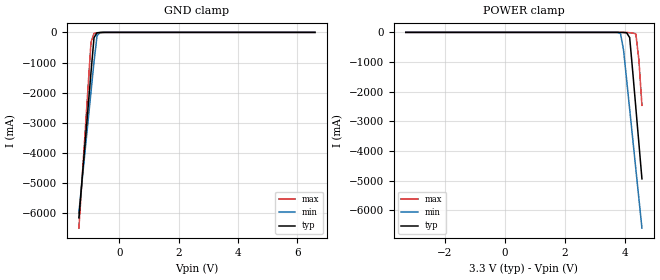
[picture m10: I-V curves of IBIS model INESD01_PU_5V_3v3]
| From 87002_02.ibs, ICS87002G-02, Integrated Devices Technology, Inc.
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[Model] INESD01_PU_5V_3v3
Model_type  Input
Polarity   Non-Inverting
Vinl = 0.8V
Vinh = 2.0V
|   typ   min   max
C_comp   2pF   1.5pF   2.5pF
|   typ   min   max
[Voltage range]  3.3V   3.15V   3.45V
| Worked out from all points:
|   GND clamp passes 1 mA (typ) near -0.55 V on its own axis
[GND_clamp]
|Voltage   I(typ)   I(min)   I(max)
-1.361V   -6.144A    -5.981A    -6.488A
-952.6mV  -1.327A    -1.975A    -329.1mA
-850.5mV  -175.3mA   -975.1mA   -32.14mA
-748.5mV  -12.69mA   -105.5mA   -18.41mA
-646.4mV  -3.879mA   -5.373mA   -8.361mA
6.6V      64.3uA     69.07uA    57.85uA
[POWER_clamp]
|Voltage   I(typ)   I(min)   I(max)
-3.3V     64.3uA     65.78uA    60.89uA
3.64V     -77.24uA   -259.7uA   -67.18uA
3.844V    -891.1uA   -31.75mA   -111uA
3.946V    -3.879mA   -592.2mA   -637.6uA
4.048V    -12.69mA   -1.591A    -3.93mA
4.151V    -175.3mA   -2.592A    -11.88mA
4.253V    -1.327A    -3.593A    -22.9mA
4.355V    -2.53A     -4.595A    -47.73mA
4.457V    -3.735A    -5.597A    -918.9mA
4.559V    -4.939A    -6.6A      -2.458A
